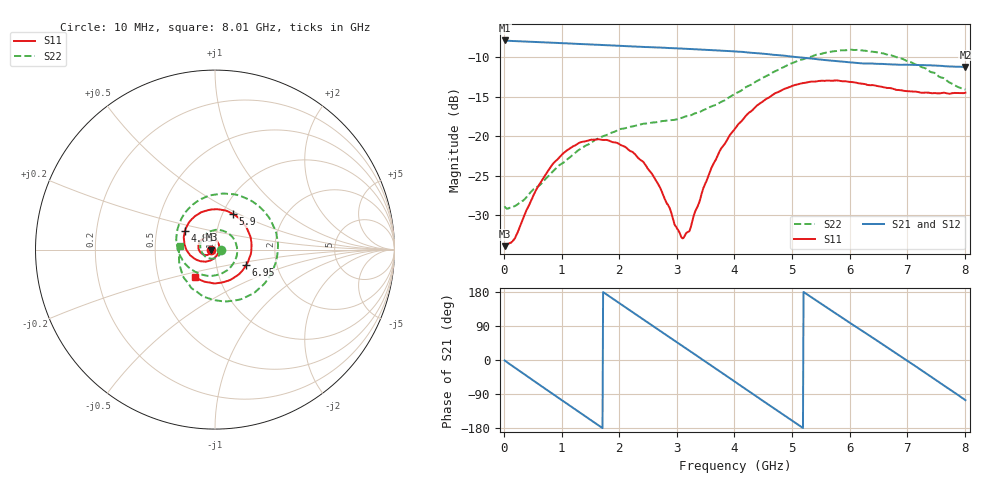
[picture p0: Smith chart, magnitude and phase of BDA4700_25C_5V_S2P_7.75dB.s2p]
!Agilent Technologies,E5071B,MY42404982,A.09.10
!Date: Mon Oct 20 13:29:52 2025
!Data & Calibration Information:
!Freq	S11:SOLT2(ON)	S21:SOLT2(ON)	S12:SOLT2(ON)	S22:SOLT2(ON)
# Hz S RI R 50
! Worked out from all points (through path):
!   801 points, 10 MHz to 8.01 GHz, reference 50 ohm
!   highest |S21| = -7.86 dB at 10 MHz (marker M1); lowest = -11.2 dB at 8.01 GHz (marker M2)
!   group delay of S21, straight-line fit = 286 ps
!   lowest |S11| = -33.9 dB at 10 MHz (marker M3), VSWR 1.04, Z = 48 - j0.0818 ohm
!   |S11| at or under -10 dB: start of sweep to end of sweep
!   |S22| runs from -29.2 to -9.0 dB; largest |S21 - S12| = 0.0031
!   S11 on the Smith chart (normalised r, x): 10 MHz: 0.96, -0.00; 4.83 GHz: 0.70, +0.15; 5.9 GHz: 1.11, +0.47; 6.95 GHz: 1.39, -0.25; 8.01 GHz: 0.77, -0.24
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1e7  -0.0201 -0.000851  0.4043 -0.00877  0.4042 -0.00911  0.0358 -0.00274
2e8  -0.0208 -0.01  0.3723 -0.1469  0.3722 -0.1473  0.0311 -0.0187
7.1e8  -0.0471 -0.0306  0.0997 -0.3804  0.0996 -0.3804  -0.0156 -0.0508
1.02e9  -0.074 -0.0225  -0.1185 -0.37  -0.1187 -0.3702  -0.0578 -0.035
1.35e9  -0.0918 0.00474  -0.3032 -0.2349  -0.3035 -0.235  -0.0821 0.0178
1.64e9  -0.0884 0.0363  -0.376 -0.0501  -0.3762 -0.0501  -0.0643 0.0724
1.93e9  -0.0673 0.0615  -0.3464 0.1437  -0.3465 0.1439  -0.00958 0.1067
2.32e9  -0.0248 0.069  -0.1685 0.3286  -0.1684 0.3287  0.0793 0.0867
2.68e9  0.0109 0.048  0.0634 0.3593  0.0632 0.3592  0.1232 0.00533
3.12e9  0.022 -0.00571  0.2953 0.2034  0.2951 0.2038  0.0802 -0.1052
3.23e9  0.0173 -0.019  0.3281 0.1412  0.3283 0.1407  0.0545 -0.1235
3.55e9  -0.0141 -0.0542  0.3473 -0.0596  0.3474 -0.0607  -0.0396 -0.146
4.01e9  -0.0938 -0.0605  0.1852 -0.2906  0.1854 -0.2903  -0.1693 -0.0751
4.4e9  -0.1571 -0.00576  -0.0464 -0.3326  -0.0463 -0.3331  -0.2159 0.0617
4.83e9  -0.168 0.1019  -0.2574 -0.1979  -0.2565 -0.1986  -0.1474 0.2281
5.35e9  -0.0703 0.2102  -0.2984 0.084  -0.2987 0.0834  0.0831 0.31
5.9e9  0.0984 0.2  -0.0943 0.2809  -0.0947 0.2805  0.314 0.1546
6.27e9  0.1783 0.1178  0.0891 0.2748  0.0914 0.2737  0.3455 -0.0417
6.68e9  0.2019 -0.0101  0.246 0.1449  0.2464 0.1446  0.2387 -0.2239
6.95e9  0.1725 -0.0875  0.2832 0.0172  0.2832 0.0157  0.1155 -0.2826
7.54e9  0.0254 -0.1852  0.1514 -0.235  0.151 -0.2354  -0.1468 -0.1906
8.01e9  -0.1096 -0.1533  -0.0754 -0.2637  -0.0755 -0.264  -0.1962 0.0211
